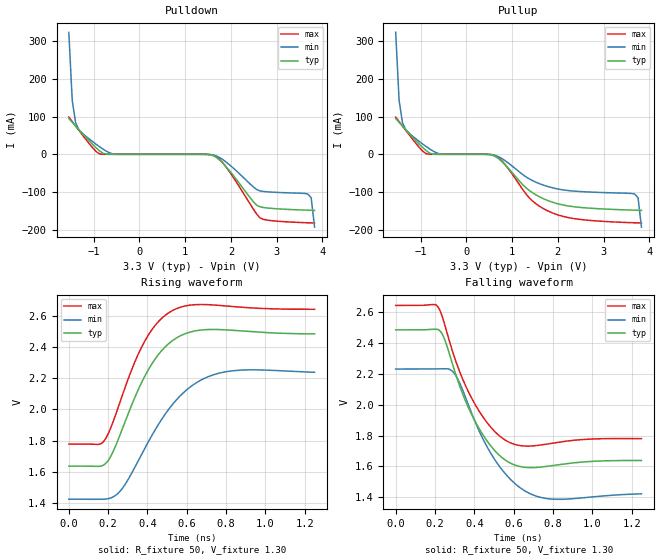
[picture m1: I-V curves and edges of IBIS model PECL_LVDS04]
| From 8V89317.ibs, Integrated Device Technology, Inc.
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|   Model lvpecl
[Model]   PECL_LVDS04
Model_type   Output_ECL
Polarity   Non-Inverting
|   typ   min   max
C_comp   2pF   1.5pF   2.5pF
Vmeas = 2.08V
Rref = 50
Cref = 0
Vref = 1.3V
|   typ   min   max
[Voltage range]   3.3V   3.135V   3.465V
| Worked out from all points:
|   rising waveform, R_fixture 50, V_fixture 1.30: 20-80 % time 183ps typ, 239ps min, 167ps max; typ from 1.64 V to 2.48 V
|   falling waveform, R_fixture 50, V_fixture 1.30: 20-80 % time 166ps typ, 189ps min, 167ps max; typ from 2.48 V to 1.64 V
[Pulldown]
|Voltage   I (typ)   I (min)   I (max)
|Note, modeling breaks down at 250mA and above.  This is well beyond the functional   |
|operating range of the device.  Should this scenario occur, catastrophic failure and   |
|possible damage to the device and/or board is of higher concern than the I-V curve   |
|behavior.  The IBIS checker will flag currents in excess of 10A with warnings.  Lines   |
|with currents in excess of 0.35 A have been commented out.  The points still remain|
|available to the user if the user desires to use them.   |
|-3.04000e+00   8.13628e+00   7.40568e+00   9.05264e+00
|-2.78000e+00   6.48842e+00   6.17138e+00   6.94615e+00
|-2.52000e+00   4.84065e+00   4.93719e+00   4.83974e+00
|-2.26000e+00   3.19294e+00   3.70309e+00   2.73339e+00
|-2.00000e+00   1.54529e+00   2.46908e+00   6.27077e-01
|-1.99000e+00   1.48192e+00   2.42162e+00   5.48040e-01
|-1.91540e+00   1.00920e+00   2.06758e+00   1.98610e-01
|-1.84080e+00   5.37180e-01   1.71354e+00   1.48402e-01
|-1.76621e+00   2.09338e-01   1.35951e+00   1.34910e-01
|-1.69161e+00   1.23802e-01   1.00548e+00   1.22822e-01
|-1.61701e+00   1.05710e-01   6.51459e-01   1.10791e-01
-1.542V   94.94mA    323.2mA    98.78mA
-1.468V   84.75mA    142.9mA    86.78mA
-1.393V   74.65mA    83.42mA    74.82mA
-1.095V   35.36mA    40.48mA    28.07mA
-871mV    9.149mA    20.06mA    1.232mA
-572.6mV  4.108uA    982.2uA    950.7nA
1.665V    -6.941mA   -3.619mA   -4.645mA
1.964V    -42.69mA   -27.19mA   -45.05mA
2.635V    -138.9mA   -96.87mA   -168.4mA
3.679V    -147.9mA   -105.1mA   -181.4mA
3.754V    -148.2mA   -115mA     -181.7mA
3.829V    -148.6mA   -193mA     -182mA
| 3.90322e+00   -1.49228e-01   -8.48432e-01   -1.82298e-01
| 3.97782e+00   -1.50944e-01   -2.34373e+00   -1.82574e-01
| 4.05241e+00   -1.56521e-01   -3.83983e+00   -1.82884e-01
| 4.12701e+00   -2.02437e-01   -5.33650e+00   -1.83452e-01
| 4.20161e+00   -9.28214e-01   -6.83362e+00   -1.85046e-01
| 4.27621e+00   -2.92725e+00   -8.33107e+00   -1.88918e-01
| 4.35080e+00   -4.92706e+00   -9.82879e+00   -2.02110e-01
| 4.42540e+00   -6.92744e+00   -1.13267e+01   -4.86879e-01
| 4.50000e+00   -8.92826e+00   -1.28248e+01   -2.83371e+00
| 4.51000e+00   -9.19650e+00   -1.30256e+01   -3.17645e+00
| 4.92800e+00   -2.04120e+01   -2.14217e+01   -1.75120e+01
| 5.34600e+00   -3.16289e+01   -2.98181e+01   -3.18527e+01
| 5.76400e+00   -4.28445e+01   -3.82136e+01   -4.61922e+01
| 6.18200e+00   -5.40593e+01   -4.66077e+01   -6.05302e+01
| 6.60000e+00   -6.52756e+01   -5.50006e+01   -7.48692e+01
[Pullup]
|Voltage   I (typ)   I (min)   I (max)
|Note, modeling breaks down at 250mA and above.  This is well beyond the functional   |
|operating range of the device.  Should this scenario occur, catastrophic failure and   |
|possible damage to the device and/or board is of higher concern than the I-V curve   |
|behavior.  The IBIS checker will flag currents in excess of 10A with warnings.  Lines   |
|with currents in excess of 0.35 A have been commented out.  The points still remain|
|available to the user if the user desires to use them.   |
|-3.04000e+00   8.13628e+00   7.40568e+00   9.05264e+00
|-2.78000e+00   6.48842e+00   6.17138e+00   6.94615e+00
|-2.52000e+00   4.84065e+00   4.93719e+00   4.83974e+00
|-2.26000e+00   3.19294e+00   3.70309e+00   2.73339e+00
|-2.00000e+00   1.54529e+00   2.46908e+00   6.27077e-01
|-1.99000e+00   1.48192e+00   2.42162e+00   5.48040e-01
|-1.91540e+00   1.00920e+00   2.06758e+00   1.98610e-01
|-1.84080e+00   5.37180e-01   1.71354e+00   1.48402e-01
|-1.76621e+00   2.09338e-01   1.35951e+00   1.34910e-01
|-1.69161e+00   1.23802e-01   1.00548e+00   1.22822e-01
|-1.61701e+00   1.05710e-01   6.51459e-01   1.10791e-01
-1.542V   94.94mA    323.2mA    98.78mA
-1.468V   84.75mA    142.9mA    86.78mA
-1.393V   74.65mA    83.42mA    74.82mA
-1.095V   35.36mA    40.48mA    28.07mA
-871mV    9.149mA    20.06mA    1.232mA
-572.6mV  4.135uA    982.3uA    950.9nA
620.9mV   -4.811mA   -2.487mA   -2.686mA
1.441V    -101.4mA   -69.34mA   -123mA
1.964V    -129.9mA   -90.95mA   -159mA
3.679V    -148mA     -105.2mA   -181.5mA
3.754V    -148.3mA   -115.1mA   -181.8mA
3.829V    -148.6mA   -193.1mA   -182.1mA
| 3.90322e+00   -1.49284e-01   -8.48518e-01   -1.82336e-01
| 3.97782e+00   -1.50988e-01   -2.34381e+00   -1.82600e-01
| 4.05241e+00   -1.56557e-01   -3.83989e+00   -1.82901e-01
| 4.12701e+00   -2.02464e-01   -5.33656e+00   -1.83462e-01
| 4.20161e+00   -9.28235e-01   -6.83367e+00   -1.85048e-01
| 4.27621e+00   -2.92726e+00   -8.33112e+00   -1.88915e-01
| 4.35080e+00   -4.92707e+00   -9.82883e+00   -2.02102e-01
| 4.42540e+00   -6.92745e+00   -1.13267e+01   -4.86867e-01
| 4.50000e+00   -8.92826e+00   -1.28248e+01   -2.83369e+00
| 4.51000e+00   -9.19650e+00   -1.30257e+01   -3.17644e+00
| 4.92800e+00   -2.04120e+01   -2.14217e+01   -1.75119e+01
| 5.34600e+00   -3.16288e+01   -2.98182e+01   -3.18526e+01
| 5.76400e+00   -4.28444e+01   -3.82136e+01   -4.61920e+01
| 6.18200e+00   -5.40590e+01   -4.66077e+01   -6.05298e+01
| 6.60000e+00   -6.52749e+01   -5.50006e+01   -7.48682e+01
[Ramp]
|   typ   min   max
dV/dt_r   0.525/0.194n   0.496/0.247n   0.537/0.177n
dV/dt_f   0.537/0.183n   0.507/0.204n   0.549/0.185n
R_load =   50.0000
[Rising Waveform]
R_fixture = 50
V_fixture = 1.30   | VCC_typ - 2V
V_fixture_max = 1.465   | VCC_max - 2V
V_fixture_min = 1.135   | VCC_min - 2V
C_fixture = 0.0p
| Time   typ   min   max
0s        1.637V     1.426V     1.779V
180.2ps   1.647V     1.426V     1.8V
216.5ps   1.708V     1.435V     1.892V
266.5ps   1.856V     1.485V     2.07V
376.6ps   2.188V     1.728V     2.414V
446.7ps   2.336V     1.886V     2.549V
524.3ps   2.437V     2.027V     2.63V
639.4ps   2.501V     2.163V     2.67V
772ps     2.51V      2.234V     2.665V
1.25ns    2.483V     2.237V     2.64V
[Falling Waveform]
R_fixture = 50
V_fixture = 1.30   | VCC_typ - 2V
V_fixture_max = 1.465   | VCC_max - 2V
V_fixture_min = 1.135   | VCC_min - 2V
C_fixture = 0.0p
| Time   typ   min   max
0s        2.483V     2.23V      2.641V
207.7ps   2.487V     2.231V     2.642V
242.7ps   2.44V      2.232V     2.545V
289ps     2.262V     2.215V     2.344V
349.1ps   2.042V     2.067V     2.14V
416.7ps   1.862V     1.851V     1.973V
568.1ps   1.632V     1.538V     1.762V
663.2ps   1.594V     1.437V     1.732V
769.5ps   1.601V     1.392V     1.745V
1.25ns    1.638V     1.423V     1.78V
